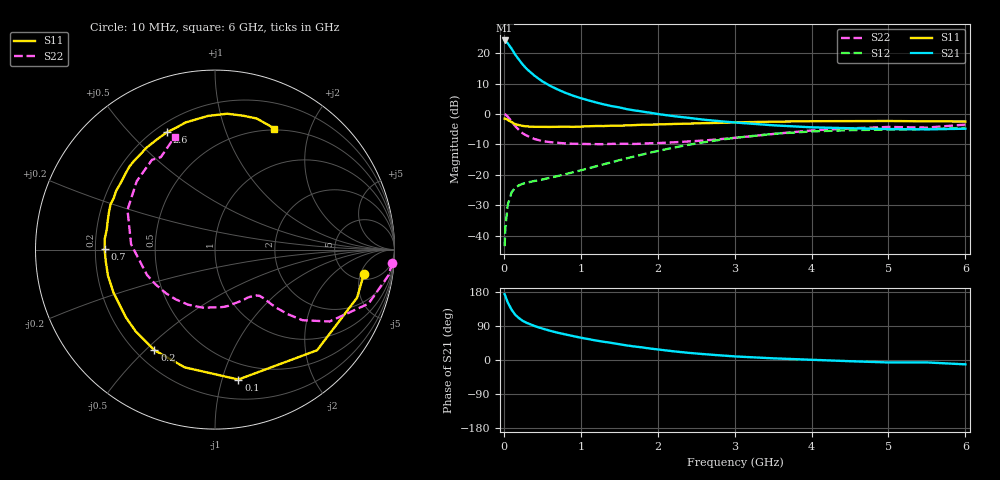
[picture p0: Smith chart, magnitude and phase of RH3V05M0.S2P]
! SIEMENS Small Signal Semiconductors
! BFR106
! Si NPN RF Bipolar Junction Transistor in SOT23
! VCE = 3 V  IC = 5 mA
! Common Emitter S-Parameters:  August  1996
# GHz  S  MA  R  50
!  f  S11  S21  S12  S22
! GHz  MAG  ANG  MAG  ANG  MAG  ANG  MAG  ANG
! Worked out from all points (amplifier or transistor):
!   36 points, 10 MHz to 6 GHz, reference 50 ohm
!   highest |S21| = 24.2 dB at 10 MHz (marker M1)
!   |S21| within 3 dB of that: start of sweep to 107.7 MHz
!   unconditionally stable (mu >= 1): 613.3 MHz to 2.068 GHz; 4.51 GHz to end of sweep
!   at 250 MHz: K = 0.51, MSG = 19.5 dB, |S12| = -22.9 dB
!   at 1.4 GHz: K = 1.15, MAG = 6.9 dB, |S12| = -15.9 dB
!   at 6 GHz: K = 1.02, MAG = -1.1 dB, |S12| = -4.6 dB
!   S11 on the Smith chart (normalised r, x): 10 MHz: 6.11, -5.71; 100 MHz: 0.36, -1.13; 200 MHz: 0.27, -0.53; 700 MHz: 0.24, +0.00; 2.6 GHz: 0.25, +0.64; 6 GHz: 0.48, +1.50
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0.01  0.8404 -9.4  16.16 173.6  0.0067 86.8  0.9906 -4.2
0.02  0.8358 -18.7  15.87 168.6  0.0136 82.8  0.9775 -8.4
0.05  0.7987 -44.6  14.54 152.3  0.0317 67.1  0.9069 -19.4
0.1  0.7354 -79.8  11.86 133.0  0.0513 53.7  0.7538 -32.1
0.15  0.6775 -104.4  9.388 118.9  0.0618 44.0  0.6264 -38.9
0.2  0.6542 -121.1  7.706 110.0  0.0674 40.2  0.5407 -41.6
0.25  0.6347 -134.1  6.398 102.8  0.0715 37.9  0.4759 -43.3
0.3  0.6237 -142.8  5.465 97.8  0.0745 37.5  0.4385 -44.1
0.4  0.6144 -156.9  4.243 89.7  0.0791 37.9  0.3862 -44.9
0.5  0.6138 -166.3  3.439 83.0  0.0836 40.2  0.3581 -46.0
0.6  0.6121 -173.9  2.907 77.2  0.0893 42.8  0.3447 -47.9
0.7  0.615 179.8  2.528 72.0  0.0953 45.7  0.3361 -50.6
0.9  0.6134 169.4  1.999 63.1  0.11 51.1  0.3234 -56.1
1.1  0.6273 160.2  1.673 55.1  0.1276 55.4  0.3202 -63.9
1.6  0.6482 142.1  1.199 38.4  0.1864 60.0  0.3229 -85.7
2.2  0.684 123.9  0.923 23.1  0.278 56.6  0.3414 -116.1
2.6  0.7065 112.4  0.805 15.5  0.3423 50.9  0.3659 -138.3
3.5  0.7461 92.9  0.651 4.4  0.4704 34.2  0.4684 176.4
4.5  0.7623 78.2  0.582 -3.2  0.5406 15.2  0.579 138.9
5  0.7665 72.4  0.565 -6.5  0.5554 7.6  0.6113 125.1
5.5  0.7558 67.3  0.558 -6.4  0.5642 3.8  0.5969 120.4
6  0.7508 63.8  0.572 -11.5  0.5897 -3.9  0.6682 109.5
